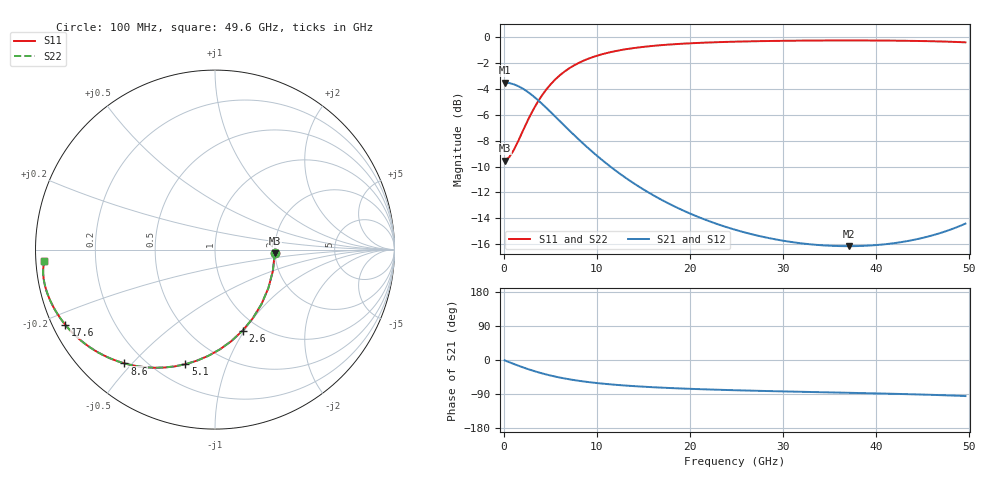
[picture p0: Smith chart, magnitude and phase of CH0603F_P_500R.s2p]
# GHz S RI R 500
! S-Parameters data
! Freq  reS11  imS11  reS21  imS21  reS12  imS12  reS22  imS22
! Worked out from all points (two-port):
!   100 points, 100 MHz to 49.6 GHz, reference 500 ohm
!   highest |S21| = -3.52 dB at 100 MHz (marker M1); lowest = -16.1 dB at 37.1 GHz (marker M2)
!   |S21| within 3 dB of the highest: start of sweep to 6.069 GHz
!   lowest |S11| = -9.5 dB at 100 MHz (marker M3), VSWR 2.00, Z = 998 - j45.2 ohm
!   |S11| at or under -10 dB: nowhere
!   |S22| runs from -9.5 to -0.3 dB; largest |S21 - S12| = 0
!   S11 on the Smith chart (normalised r, x): 100 MHz: 2.00, -0.09; 2.6 GHz: 0.84, -0.98; 5.1 GHz: 0.32, -0.72; 8.6 GHz: 0.13, -0.48; 17.6 GHz: 0.04, -0.24; 49.6 GHz: 0.02, -0.03
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0.1  0.333 -0.0201  0.6665 -0.0113  0.6665 -0.0113  0.333 -0.0201
0.6  0.3223 -0.1197  0.6601 -0.0671  0.6601 -0.0671  0.3223 -0.1197
1.1  0.2971 -0.2153  0.6449 -0.1203  0.6449 -0.1203  0.2971 -0.2153
2.1  0.2102 -0.3831  0.5935 -0.2119  0.5935 -0.2119  0.2102 -0.3831
2.6  0.1535 -0.4519  0.5606 -0.2482  0.5606 -0.2482  0.1535 -0.4519
3.6  0.0269 -0.5561  0.4885 -0.3008  0.4885 -0.3008  0.0269 -0.5561
4.1  -0.0385 -0.5925  0.4521 -0.3179  0.4521 -0.3179  -0.0385 -0.5925
5.1  -0.1653 -0.6386  0.3835 -0.3373  0.3835 -0.3373  -0.1653 -0.6386
6.6  -0.3326 -0.6584  0.2966 -0.3409  0.2966 -0.3409  -0.3326 -0.6584
8.6  -0.5042 -0.634  0.2122 -0.3224  0.2122 -0.3224  -0.5042 -0.634
10.1  -0.5991 -0.5994  0.1677 -0.3028  0.1677 -0.3028  -0.5991 -0.5994
12.1  -0.692 -0.5476  0.1256 -0.2765  0.1256 -0.2765  -0.692 -0.5476
14.1  -0.7579 -0.4972  0.0966 -0.2528  0.0966 -0.2528  -0.7579 -0.4972
16.6  -0.8154 -0.4405  0.0719 -0.2281  0.0719 -0.2281  -0.8154 -0.4405
17.6  -0.833 -0.42  0.0644 -0.2197  0.0644 -0.2197  -0.833 -0.42
21.1  -0.8783 -0.3574  0.0452 -0.1957  0.0452 -0.1957  -0.8783 -0.3574
25.1  -0.9105 -0.2999  0.0313 -0.1767  0.0313 -0.1767  -0.9105 -0.2999
33.1  -0.9438 -0.2133  0.0152 -0.1576  0.0152 -0.1576  -0.9438 -0.2133
37.1  -0.9521 -0.1777  0.00931 -0.1557  0.00931 -0.1557  -0.9521 -0.1777
41.6  -0.9569 -0.1395  0.00262 -0.1596  0.00262 -0.1596  -0.9569 -0.1395
45.6  -0.9568 -0.104  -0.00499 -0.1699  -0.00499 -0.1699  -0.9568 -0.104
49.6  -0.9504 -0.0628  -0.0172 -0.1897  -0.0172 -0.1897  -0.9504 -0.0628
